(* 	
	Program Name: 	ACS_CMD_DISABLE
	Purpose:		Copy Disable Command to ACS Drive Output Command Register
	When Executed:	Disables motor power to drive
*)
PROGRAM ACS_CMD_DISABLE
VAR_IN_OUT
	Axis:ACS_DRIVE_TYPE;
END_VAR
VAR
	_command:	USINT	:= ACS_COMMANDS.DISABLE;
END_VAR

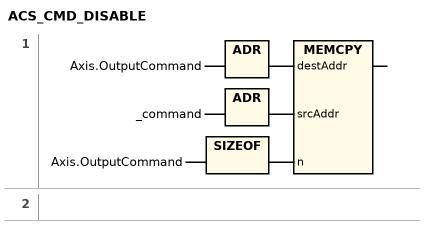
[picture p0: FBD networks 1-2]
// NETWORK 1
MEMCPY(destAddr := ADR(Axis.OutputCommand), srcAddr := ADR(_command), n := SIZEOF(Axis.OutputCommand));

// NETWORK 2

END_PROGRAM
